PROGRAM MAIN_SLOW
VAR
	iAxis                : USINT;  (* Axis index *)
	configurationManager : ConfigurationManager;  (* The axis configuration FB *)
	twincatEventTrialink : TL_TwinCatError;  (* Axis independent events of the library *)

END_VAR

(* ------------------------------------------- *)
(* Triamec Motion AG, 6340 Baar, Switzerland   *)
(* Sample Code may be adapted to customer need *)
(* ------------------------------------------- *)

configurationManager();
gTrialink.CallSlow();

IF NOT gHli.Initialized THEN
	gHli();			(* initialize HLI *)
END_IF

gCommunicationReady	:= NOT gTrialink.error;
FOR iAxis:=1 TO N_AXES DO

	gAxes[iAxis].iAxis	:= iAxis;	(* logical axis number used in MAIN_FAST *)
	gAxes[iAxis].reset	:= gReset;	(* reset drive errors *)
	gAxes[iAxis].enable	:= gEnable;	(* set enable/disable *)
	gAxes[iAxis].couple	:= TRUE;	(* couple drive to CNC-pathplanner *)
	gAxes[iAxis].CallSlow( Trialink := gTrialink );

	gCommunicationReady	:= gCommunicationReady 	AND gAxes[iAxis].ready;

	gCncAxes[iAxis].CommunicationReady	:= gAxes[iAxis].ready;
	gCncAxes[iAxis].ReleaseFeedhold		:= gAxes[iAxis].enabled;
	gCncAxes[iAxis].TorquePermission	:= gAxes[iAxis].coupled;
	gCncAxes[iAxis].AxisTracking		:= gAxes[iAxis].followMe;
	gCncAxes[iAxis].HomingDone			:= gAxes[iAxis].referenced;
	gCncAxes[iAxis].CallSlow( axis := gAxes[iAxis].MC_axis);

END_FOR

// Sample code to asynchronously read any drive register
motorTemperature1.Execute		:= TRUE; // Toggle to restart reading
motorTemperature1.SetReg		:= gAxes[1].MC_Axis.register2.Axis.Signals.General.MotorTemperature;
motorTemperature1(axis := gAxes[1].MC_axis, Trialink := gTrialink);

// Sample code to cyclically read four drive registers
publish1.src1 := gAxes[1].MC_axis.register2.Axis.Signals.CurrentController.ActualCurrentQ;
publish1.src2 := gAxes[1].MC_axis.register2.Axis.Signals.CurrentController.ActualCurrentQ;
publish1.src3 := gAxes[1].MC_axis.register2.Axis.Signals.CurrentController.ActualCurrentQ;
publish1.src4 := gAxes[1].MC_axis.register2.Axis.Signals.CurrentController.ActualCurrentQ;
publish1.station := gAxes[1].MC_axis.station;
publish1.CallSlow(Trialink := gTrialink);

// Sample code to throw Trialink errors as a TwinCAT event
twincatEventTrialink.Execute	:= gTrialink.Error;
twincatEventTrialink.errorId	:= gTrialink.ErrorId;
twincatEventTrialink.source		:= TL_EventSourceId.Trialink; // See source entry in the ecpx file triamecEventsTrialinkLib*.ecpx
twincatEventTrialink.par1		:= UDINT_TO_DINT(gTrialink.Config.nDevId);
twincatEventTrialink();

END_PROGRAM
